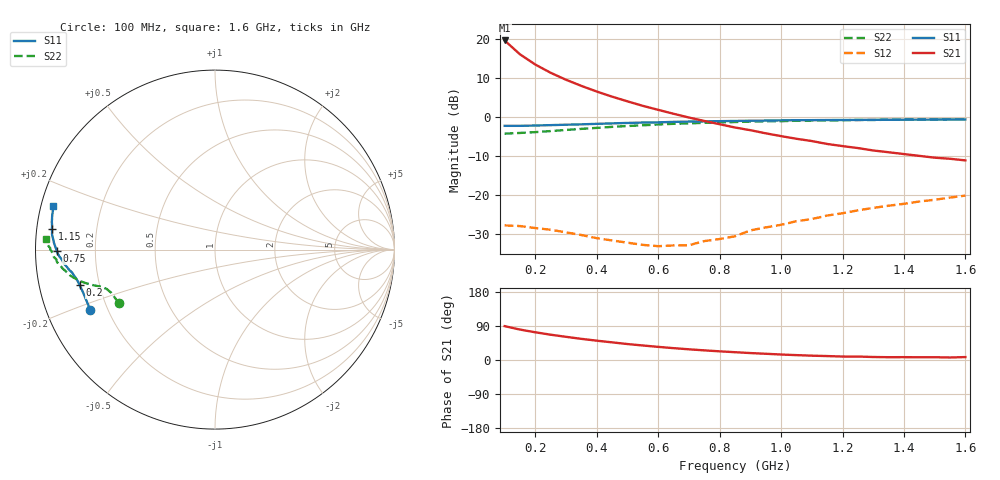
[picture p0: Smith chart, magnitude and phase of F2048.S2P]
! Date: Mon Aug 14 14:28:17 1995
# MHZ  S  MA  R  50.0000
!  POLYFET RF DEVICES
!  F2048
!  S PARAMETERS
!  VDS=28V, IDQ=800mA
! FREQ  S11MAG  S11ANG  S21MAG  S21ANG  S12MAG  S12ANG  S22MAG  S22ANG
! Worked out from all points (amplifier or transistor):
!   31 points, 100 MHz to 1.6 GHz, reference 50 ohm
!   highest |S21| = 19.7 dB at 100 MHz (marker M1)
!   |S21| within 3 dB of that: start of sweep to 142.2 MHz
!   unconditionally stable (mu >= 1): 495.1 MHz to 858.4 MHz
!   at 350 MHz: K = 0.67, MSG = 19.1 dB, |S12| = -30.3 dB
!   at 850 MHz: K = 1.04, MAG = 12.7 dB, |S12| = -30.6 dB
!   at 1.6 GHz: K = 0.36, MSG = 4.5 dB, |S12| = -20.1 dB
!   S11 on the Smith chart (normalised r, x): 100 MHz: 0.14, -0.23; 200 MHz: 0.13, -0.13; 750 MHz: 0.06, -0.00; 1.15 GHz: 0.04, +0.06; 1.6 GHz: 0.04, +0.13
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100  0.772 -154.0  9.611 89.4  0.04081 7.3  0.6131 -150.9
150  0.7723 -161.6  6.383 80.3  0.04002 2.0  0.6258 -157.3
200  0.7793 -165.4  4.719 73.1  0.03774 -0.6  0.6415 -160.0
250  0.7882 -167.9  3.698 66.7  0.03589 -2.5  0.6615 -161.6
300  0.7986 -169.6  3.009 61.1  0.03324 -3.2  0.6839 -162.7
350  0.8066 -170.9  2.512 55.8  0.03071 -2.3  0.706 -163.7
400  0.8196 -172.0  2.126 51.0  0.02798 0.9  0.7271 -164.7
450  0.83 -173.3  1.828 46.6  0.02615 4.1  0.7491 -165.7
500  0.841 -174.3  1.592 42.1  0.0245 9.1  0.7682 -166.7
550  0.8508 -175.5  1.393 38.3  0.02295 16.2  0.7847 -167.7
600  0.8558 -176.4  1.239 34.7  0.0221 26.0  0.8033 -168.8
650  0.8681 -177.5  1.103 31.2  0.02259 31.4  0.82 -169.9
700  0.8758 -178.5  0.9869 28.2  0.02271 41.1  0.8312 -171.0
750  0.8806 -179.5  0.8921 25.4  0.02567 47.9  0.8443 -172.1
850  0.8923 178.6  0.7352 20.6  0.02961 62.5  0.8638 -173.8
900  0.8982 177.5  0.6788 18.3  0.03522 64.5  0.8767 -174.8
1000  0.9078 175.6  0.5699 14.5  0.04154 68.6  0.8859 -176.5
1050  0.912 174.7  0.5269 12.9  0.04617 69.9  0.8982 -177.3
1100  0.9133 173.6  0.4929 11.4  0.0492 71.0  0.9023 -178.1
1150  0.9165 172.7  0.452 10.4  0.05459 71.1  0.9056 -178.8
1350  0.924 169.3  0.3541 7.4  0.07299 71.9  0.9258 178.9
1600  0.9326 165.0  0.2783 7.7  0.09842 68.3  0.9408 176.4
